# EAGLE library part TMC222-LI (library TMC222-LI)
Micro Stepping Stepper Motor Controller / Driver with Two Wire Serial Interface, QFN32(7x7)
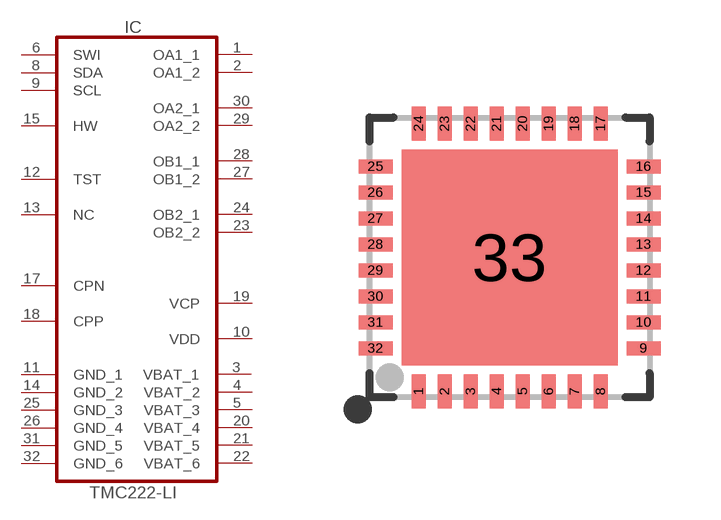
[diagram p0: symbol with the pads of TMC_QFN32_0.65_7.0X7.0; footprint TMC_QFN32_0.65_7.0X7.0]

Designator prefix IC

## TMC222-LI (DATASHEET: http://www_trinamic_com/_scripts/download_php?file=_articles%2Fproducts%2Fintegrated-circuits%2Ftmc222%2F_datasheet%2FTMC222_datasheet_pdf; DESCRIPTION: Micro Stepping Stepper Motor Controller / Driver with Two Wire Serial Interface, QFN32(7x7); DISTRIBUTOR1: Digikey; DISTRIBUTOR2: Farnell; GEOMETRY_HEIGHT: 0,9mm; MANUFACTURER: TRINAMIC; ORDERCODE-DISTRI1: 1460-1051-ND; ORDERCODE-MANU1: TMC222-LI; VALUE: TMC222-LI)  [TMC_QFN32_0.65_7.0X7.0]
1  OA1_1  out
2  OA1_2  out
3  VBAT_1  pwr
4  VBAT_2  pwr
5  VBAT_3  pwr
6  SWI  in
8  SDA
9  SCL  in
10  VDD  pwr
11  GND_1  pwr
12  TST  in
13  NC  pas
14  GND_2  pwr
15  HW  in
17  CPN
18  CPP
19  VCP  pwr
20  VBAT_4  pwr
21  VBAT_5  pwr
22  VBAT_6  pwr
23  OB2_2  out
24  OB2_1  out
25  GND_3  pwr
26  GND_4  pwr
27  OB1_2  out
28  OB1_1  out
29  OA2_2  out
30  OA2_1  out
31  GND_5  pwr
32  GND_6  pwr

## Footprint TMC_QFN32_0.65_7.0X7.0 (pad centres in mm)
smd 0.35 x 0.85: 1 -2.275,-3.35; 2 -1.625,-3.35; 3 -0.975,-3.35; 4 -0.325,-3.35; 5 0.325,-3.35; 6 0.975,-3.35; 7 1.625,-3.35; 8 2.275,-3.35; 17 2.275,3.35; 18 1.625,3.35; 19 0.975,3.35; 20 0.325,3.35; 21 -0.325,3.35; 22 -0.975,3.35; 23 -1.625,3.35; 24 -2.275,3.35
smd 0.85 x 0.35: 9 3.35,-2.275; 10 3.35,-1.625; 11 3.35,-0.975; 12 3.35,-0.325; 13 3.35,0.325; 14 3.35,0.975; 15 3.35,1.625; 16 3.35,2.275; 25 -3.35,2.275; 26 -3.35,1.625; 27 -3.35,0.975; 28 -3.35,0.325; 29 -3.35,-0.325; 30 -3.35,-0.975; 31 -3.35,-1.625; 32 -3.35,-2.275
smd 5.4 x 5.4: 33 0,0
